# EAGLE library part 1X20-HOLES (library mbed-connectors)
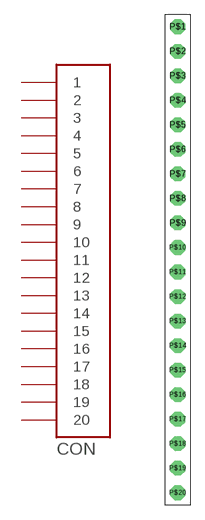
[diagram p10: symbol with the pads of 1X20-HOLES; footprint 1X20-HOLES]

Designator prefix CON

## 1X20-HOLES  [1X20-HOLES]
P$1  1
P$2  2
P$3  3
P$4  4
P$5  5
P$6  6
P$7  7
P$8  8
P$9  9
P$10  10
P$11  11
P$12  12
P$13  13
P$14  14
P$15  15
P$16  16
P$17  17
P$18  18
P$19  19
P$20  20

## Footprint 1X20-HOLES (pad centres in mm)
drill 1 octagon: P$1 0,0; P$2 0,-2.54; P$3 0,-5.08; P$4 0,-7.62; P$5 0,-10.16; P$6 0,-12.7; P$7 0,-15.24; P$8 0,-17.78; P$9 0,-20.32; P$10 0,-22.86; P$11 0,-25.4; P$12 0,-27.94; P$13 0,-30.48; P$14 0,-33.02; P$15 0,-35.56; P$16 0,-38.1; P$17 0,-40.64; P$18 0,-43.18; P$19 0,-45.72; P$20 0,-48.26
